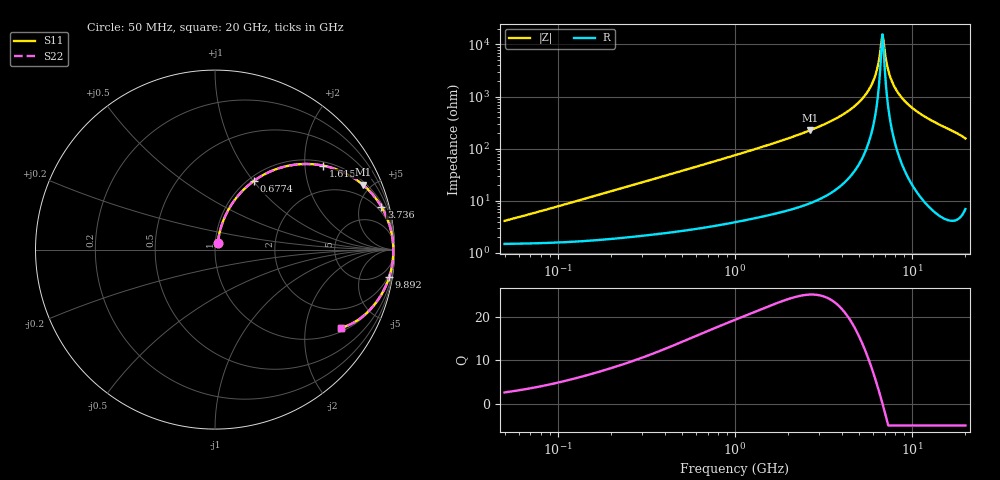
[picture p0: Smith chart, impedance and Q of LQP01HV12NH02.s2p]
!Murata Part Number: LQP01HV12NH02
!These Parameters are Measured in Series Mode Connection
!  o--[Z]--o
!Port1  Port2
!  o-------o
!Freq. Start=50[MHz] Stop=20[GHz], 401[Steps]
# Hz S RI R 50
!Freq.(Hz) S11(Real) S11(Imag) S21(Real) S21(Imag) S12(Real) S12(Imag) S22(Real) S22(Imag)
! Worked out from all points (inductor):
!   401 points, 50 MHz to 20 GHz, reference 50 ohm
!   read as one part in series: L = 12.2 nH near 58.96 MHz
!   highest Q = 25 at 2.647 GHz (marker M1), where L = 13.5 nH
!   self-resonance near 6.802 GHz
!   S11 on the Smith chart (normalised r, x): 50 MHz: 1.03, +0.08; 677.4 MHz: 1.06, +1.01; 1.615 GHz: 1.11, +2.48; 3.736 GHz: 1.33, +7.65; 9.892 GHz: 1, -13; 20 GHz: 1.14, -3.15
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5e7  0.0161 0.0374  0.9839 -0.0374  0.9839 -0.0374  0.0161 0.0374
1.364002e8  0.0268 0.0999  0.9732 -0.0999  0.9732 -0.0999  0.0268 0.0999
3.721004e8  0.0904 0.2482  0.9096 -0.2482  0.9096 -0.2482  0.0904 0.2482
6.774326e8  0.2176 0.3833  0.7824 -0.3833  0.7824 -0.3833  0.2176 0.3833
1e9  0.3661 0.4565  0.6339 -0.4565  0.6339 -0.4565  0.3661 0.4565
1.614971e9  0.6019 0.4679  0.3981 -0.4679  0.3981 -0.4679  0.6019 0.4679
2.647493e9  0.8245 0.3609  0.1755 -0.3609  0.1755 -0.3609  0.8245 0.3609
2.728004e9  0.8354 0.3514  0.1646 -0.3514  0.1646 -0.3514  0.8354 0.3514
3.736399e9  0.927 0.2392  0.073 -0.2392  0.073 -0.2392  0.927 0.2392
4.81993e9  0.9715 0.1395  0.0285 -0.1395  0.0285 -0.1395  0.9715 0.1395
5.683258e9  0.9873 0.0733  0.0127 -0.0733  0.0127 -0.0733  0.9873 0.0733
6.217679e9  0.9918 0.0369  0.00817 -0.0369  0.00817 -0.0369  0.9918 0.0369
6.406762e9  0.9927 0.0247  0.00727 -0.0247  0.00727 -0.0247  0.9927 0.0247
6.701223e9  0.9935 0.00641  0.00649 -0.00641  0.00649 -0.00641  0.9935 0.00641
6.802353e9  0.9936 0.000304  0.00639 -0.000304  0.00639 -0.000304  0.9936 0.000304
7.009217e9  0.9936 -0.0119  0.00641 0.0119  0.00641 0.0119  0.9936 -0.0119
7.222371e9  0.9933 -0.0242  0.00674 0.0242  0.00674 0.0242  0.9933 -0.0242
7.442007e9  0.9926 -0.0364  0.00739 0.0364  0.00739 0.0364  0.9926 -0.0364
8.264682e9  0.9879 -0.0794  0.0121 0.0794  0.0121 0.0794  0.9879 -0.0794
9.892087e9  0.9702 -0.1536  0.0298 0.1536  0.0298 0.1536  0.9702 -0.1536
1.504638e10  0.8712 -0.3264  0.1288 0.3264  0.1288 0.3264  0.8712 -0.3264
2e10  0.7045 -0.4347  0.2955 0.4347  0.2955 0.4347  0.7045 -0.4347
